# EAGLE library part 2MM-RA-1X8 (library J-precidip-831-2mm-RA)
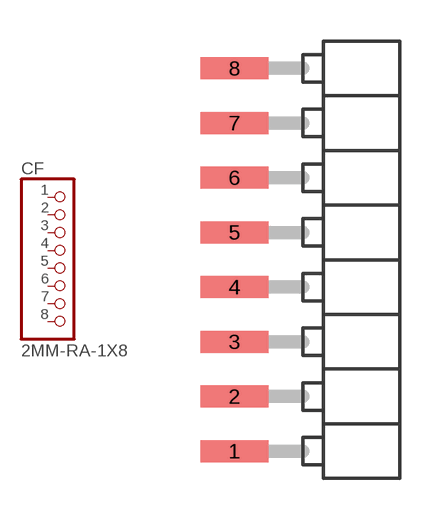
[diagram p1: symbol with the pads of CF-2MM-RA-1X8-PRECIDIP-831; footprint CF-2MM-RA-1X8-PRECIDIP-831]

Designator prefix CF

## 2MM-RA-1X8  [CF-2MM-RA-1X8-PRECIDIP-831]
1  1  pas
2  2  pas
3  3  pas
4  4  pas
5  5  pas
6  6  pas
7  7  pas
8  8  pas

## Footprint CF-2MM-RA-1X8-PRECIDIP-831 (pad centres in mm)
smd 2.5 x 0.8: 1 -3.25,-7; 2 -3.25,-5; 3 -3.25,-3; 4 -3.25,-1; 5 -3.25,1; 6 -3.25,3; 7 -3.25,5; 8 -3.25,7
